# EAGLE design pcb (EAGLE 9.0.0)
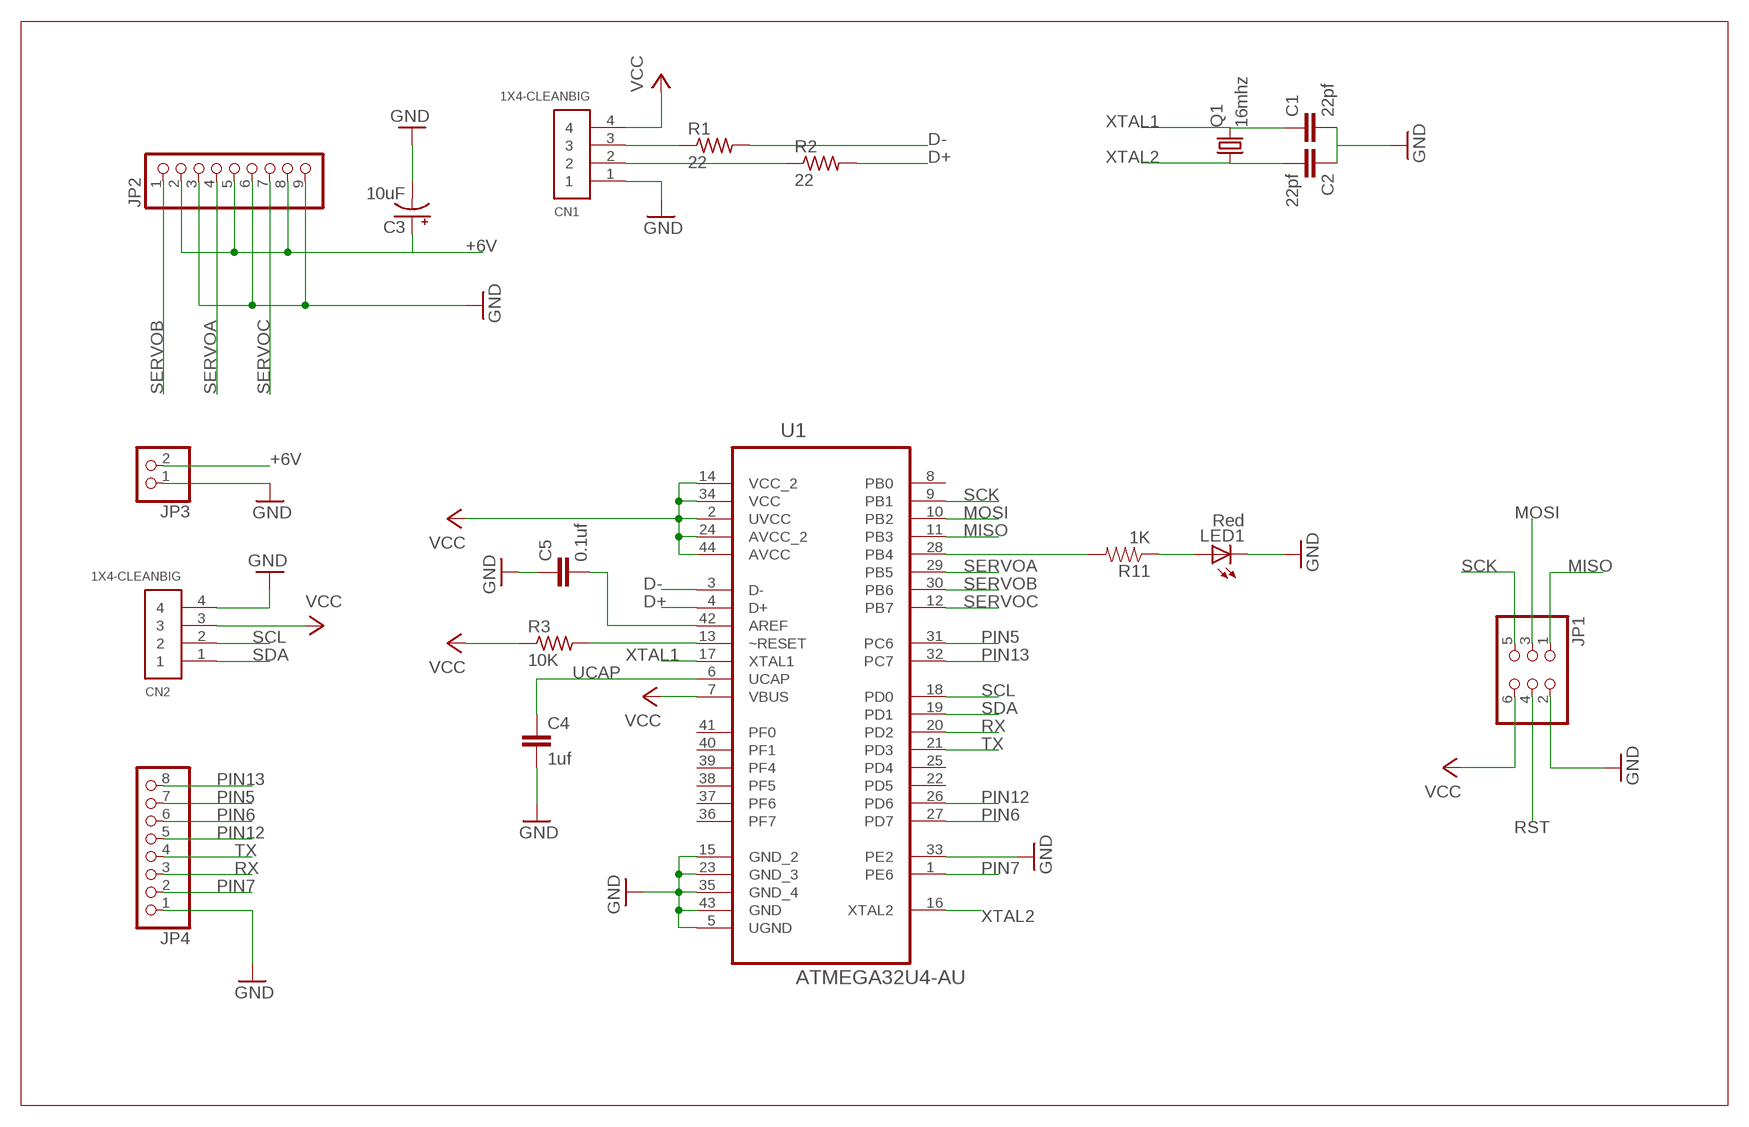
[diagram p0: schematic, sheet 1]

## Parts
C1  22pf  C5/2.5  [C5B2.5]
C2  22pf  C5/2.5  [C5B2.5]
C3  10uF  CAP_POL1206  [EIA3216]
C4  1uf  CC0603  [C0603]
C5  0.1uf  CC0603  [C0603]
CN1  1X4-CLEANBIG  [1X04-CLEANBIG]
CN2  1X4-CLEANBIG  [1X04-CLEANBIG]
JP1  PINHD-2X3  [2X03]
JP2  PINHD-1X9  [1X09-BIG]
JP3  PINHD-1X2  [1X02]
JP4  PINHD-1X8BIG  [1X08-BIG]
LED1  Red  LED0603  [LED-0603]
Q1  16mhz  CRYSTALHC49S  [HC49/S]
R1  22  R-US_R0603  [R0603]
R2  22  R-US_R0603  [R0603]
R3  10K  R-US_R0603  [R0603]
R11  1K  RESISTOR0603-RES  [0603-RES]
U1  ATMEGA32U4-AU  [QFP80P1200X1200X120-44N]

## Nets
+6V: C3.A(+) JP2.2 JP2.5 JP2.8 JP3.2
AREF: C5.2 U1.42(AREF)
D+: R2.2 U1.4(D+)
D-: R1.2 U1.3(D-)
GND: C1.2 C2.1 C3.C(-) C4.2 C5.1 CN1.1 CN2.4 JP1.2 JP2.3 JP2.6 JP2.9 JP3.1 JP4.1 LED1.C U1.5(UGND) U1.15(GND_2) U1.23(GND_3) U1.33(PE2) U1.35(GND_4) U1.43(GND)
MISO: JP1.1 U1.11(PB3)
MOSI: JP1.3 U1.10(PB2)
N$1: CN1.3 R1.1
N$2: CN1.2 R2.1
N$3: R11.2 U1.28(PB4)
N$4: LED1.A R11.1
PIN5: JP4.7 U1.31(PC6)
PIN6: JP4.6 U1.27(PD7)
PIN7: JP4.2 U1.1(PE6)
PIN12: JP4.5 U1.26(PD6)
PIN13: JP4.8 U1.32(PC7)
RST: JP1.4 R3.2 U1.13(~RESET)
RX: JP4.3 U1.20(PD2)
SCK: JP1.5 U1.9(PB1)
SCL: CN2.2 U1.18(PD0)
SDA: CN2.1 U1.19(PD1)
SERVOA: JP2.4 U1.29(PB5)
SERVOB: JP2.1 U1.30(PB6)
SERVOC: JP2.7 U1.12(PB7)
TX: JP4.4 U1.21(PD3)
UCAP: C4.1 U1.6(UCAP)
VCC: CN1.4 CN2.3 JP1.6 R3.1 U1.2(UVCC) U1.7(VBUS) U1.14(VCC_2) U1.24(AVCC_2) U1.34(VCC) U1.44(AVCC)
XTAL1: C1.1 Q1.2 U1.17(XTAL1)
XTAL2: C2.2 Q1.1 U1.16(XTAL2)
Unconnected: U1.8(PB0) U1.22(PD5) U1.25(PD4) U1.36(PF7) U1.37(PF6) U1.38(PF5) U1.39(PF4) U1.40(PF1) U1.41(PF0)

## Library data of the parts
C1 C2 = capacitor-wima:C: CAPACITOR
C3 = SparkFun:CAP_POL: Capacitor Polarized
C4 C5 = eagle-ltspice:C: CAPACITOR, European symbol; SPICEMODEL: NONE; SPICEPREFIX: C
CN1 CN2 = adafruit:1X4: 4-pin connector
JP1 = pinhead:PINHD-2X3: PIN HEADER
JP2 = adafruit:PINHD-1X9: Pin header 1x10 0.1" spacing With round pins
JP3 = pinhead:PINHD-1X2: PIN HEADER
JP4 = adafruit:PINHD-1X8: PIN HEADER
LED1 = SparkFun:LED: LEDs
Q1 = adafruit:CRYSTAL: CRYSTAL; OC_FARNELL: 1667008; OC_NEWARK: unknown
R1-R3 = adafruit:R-US_: RESISTOR, American symbol
R11 = SparkFun:RESISTOR: Resistor
U1 = ATMEGA32U4-AU:ATMEGA32U4-AU: 8-bit Microcontroller with ISP Flash and USB Controller; AVAILABILITY: Good; DESCRIPTION: MCU 8-bit ATmega AVR RISC 32KB Flash 3.3V/5V 44-Pin TQFP; MF: Microchip; MP: ATMEGA32U4-AU; PACKAGE: TQFP-44 Microchip; PRICE: 4.08 USD

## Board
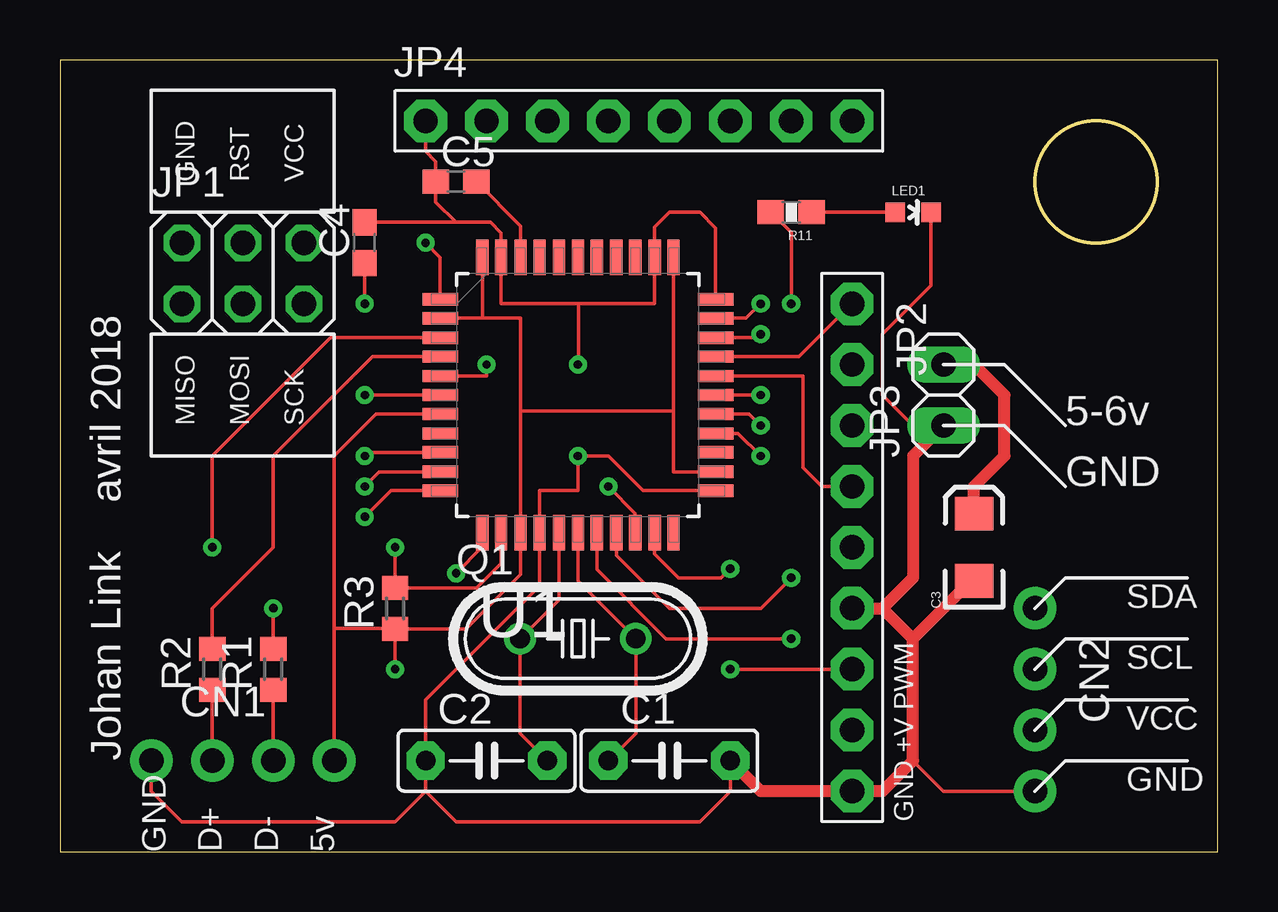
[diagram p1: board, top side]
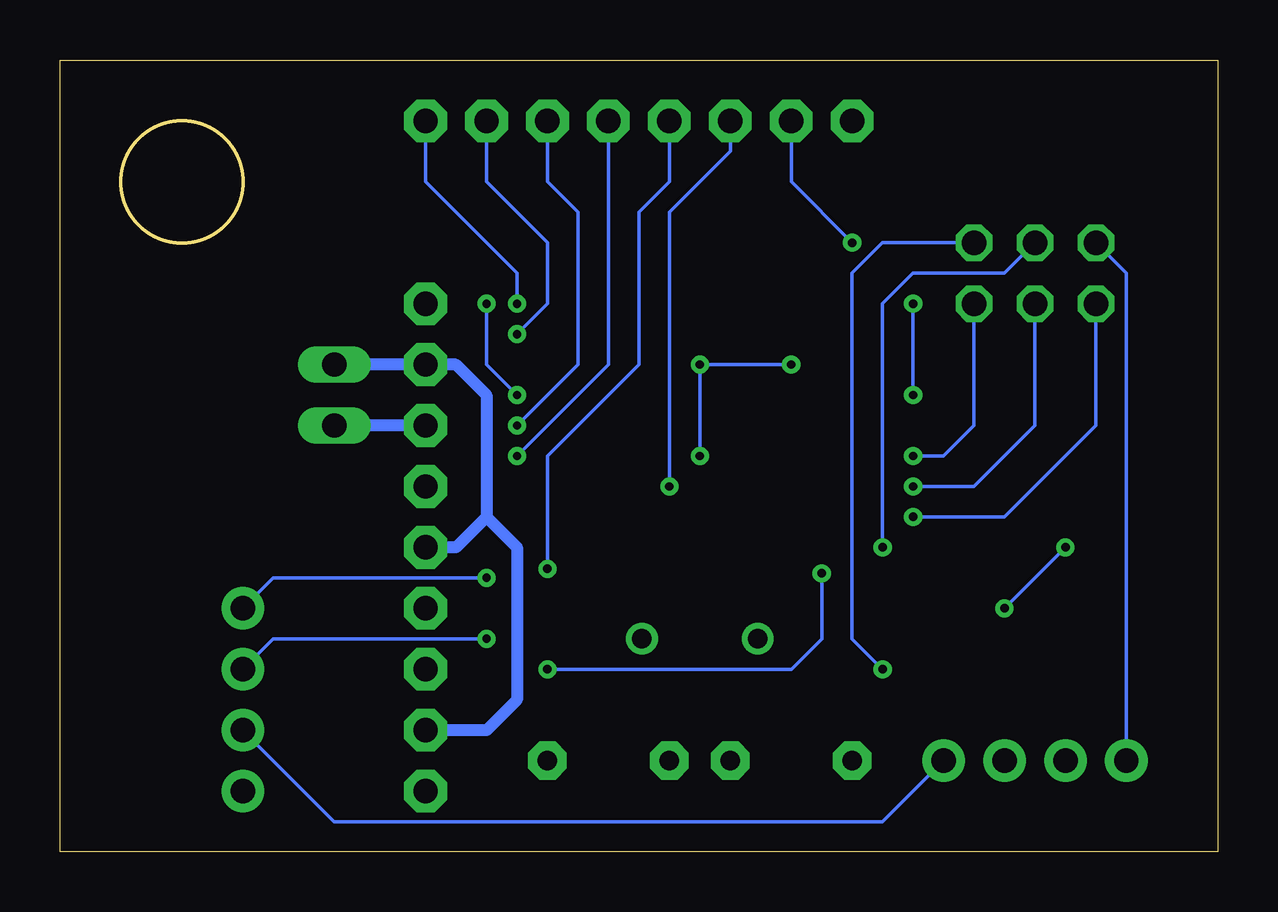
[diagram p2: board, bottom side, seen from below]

Size 48.26 x 33.02 mm. Coordinates in mm from the lower left corner, seen from the top.
Outline: 0,0 48.26,0 48.26,33.02 0,33.02 0,0
Outline: circle at 43.18,27.94 radius 2.54
Copper layers (1*16): Top 0.035mm / dielectric 1.5mm / Bottom 0.035mm
Design rules "default": minimum track width 6mil, minimum drill 0.35mm, track to track 6mil, track to pad 6mil, pad to pad 6mil, via to via 6mil, smd to smd 6mil, copper to edge 40mil, drill to drill 6mil, minimum pad ring 10mil, minimum via ring 8mil, stop-mask expansion 4mil, vias tented up to drill 0mil, thermal gap 10mil

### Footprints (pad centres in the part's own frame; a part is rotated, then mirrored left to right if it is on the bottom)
C5B2.5 = drill 0.813 pad 1.6 octagon: 1 -2.54,0; 2 2.54,0
EIA3216 = smd 1.4 x 1.6: A 1.4,0; C -1.4,0
C0603 = smd 1.1 x 1: 1 -0.85,0; 2 0.85,0
1X04-CLEANBIG = drill 1.016 pad 1.778: 1 -3.81,0; 2 -1.27,0; 3 1.27,0; 4 3.81,0
2X03 = drill 1.016 octagon: 1 -2.54,-1.27; 2 -2.54,1.27; 3 0,-1.27; 4 0,1.27; 5 2.54,-1.27; 6 2.54,1.27
1X09-BIG = drill 1.016 pad 1.778 octagon: 1 -10.16,0; 2 -7.62,0; 3 -5.08,0; 4 -2.54,0; 5 0,0; 6 2.54,0; 7 5.08,0; 8 7.62,0; 9 10.16,0
1X02 = drill 1.016 long: 1 -1.27,0; 2 1.27,0
1X08-BIG = drill 1.016 pad 1.778 octagon: 1 -8.89,0; 2 -6.35,0; 3 -3.81,0; 4 -1.27,0; 5 1.27,0; 6 3.81,0; 7 6.35,0; 8 8.89,0
LED-0603 = smd 0.8 x 0.8: A 0,-0.75; C 0,0.75
HC49/S = drill 0.813: 1 -2.413,0; 2 2.413,0
R0603 = smd 1 x 1.1: 1 -0.85,0; 2 0.85,0
0603-RES = smd 1.1 x 1: 1 -0.85,0; 2 0.85,0
QFP80P1200X1200X120-44N = smd 1.473 x 0.508: 1 -5.74,3.988; 2 -5.74,3.2; 3 -5.74,2.388; 4 -5.74,1.6; 5 -5.74,0.787; 6 -5.74,0; 7 -5.74,-0.787; 8 -5.74,-1.6; 9 -5.74,-2.388; 10 -5.74,-3.2; 11 -5.74,-3.988; 23 5.74,-3.988; 24 5.74,-3.2; 25 5.74,-2.388; 26 5.74,-1.6; 27 5.74,-0.787; 28 5.74,0; 29 5.74,0.787; 30 5.74,1.6; 31 5.74,2.388; 32 5.74,3.2; 33 5.74,3.988 | smd 0.508 x 1.473: 12 -3.988,-5.74; 13 -3.2,-5.74; 14 -2.388,-5.74; 15 -1.6,-5.74; 16 -0.787,-5.74; 17 0,-5.74; 18 0.787,-5.74; 19 1.6,-5.74; 20 2.388,-5.74; 21 3.2,-5.74; 22 3.988,-5.74; 34 3.988,5.74; 35 3.2,5.74; 36 2.388,5.74; 37 1.6,5.74; 38 0.787,5.74; 39 0,5.74; 40 -0.787,5.74; 41 -1.6,5.74; 42 -2.388,5.74; 43 -3.2,5.74; 44 -3.988,5.74

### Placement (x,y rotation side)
C1  25.4,3.81 0 top
C2  17.78,3.81 0 top
C3  38.1,12.7 90 top
C4  12.7,25.4 90 top
C5  16.51,27.94 0 top
CN1  7.62,3.81 0 top
CN2  40.64,6.35 270 top
JP1  7.62,24.13 0 top
JP2  33.02,12.7 270 top
JP3  36.83,19.05 90 top
JP4  24.13,30.48 0 top
LED1  35.56,26.67 270 top
Q1  21.59,8.89 0 top
R1  8.89,7.62 90 top
R2  6.35,7.62 90 top
R3  13.97,10.16 90 top
R11  30.48,26.67 180 top
U1  21.59,19.05 0 top

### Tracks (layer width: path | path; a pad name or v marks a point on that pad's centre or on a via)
+6V
  Top 0.508: C3.A 38.1,15.24 39.37,16.51 39.37,19.05 38.1,20.32 JP3.2
  Bottom 0.508: 30.48,13.97 30.48,19.05 31.75,20.32 JP2.2 JP3.2 | 30.48,13.97 29.21,12.7 29.21,6.35 30.48,5.08 JP2.8 | 30.48,13.97 31.75,12.7 JP2.5
AREF
  Top 0.152: C5.2 19.2,26.1 U1.42
D+
  Top 0.152: U1.4 13.03,20.65 8.89,16.51 8.89,12.7 6.35,10.16 R2.2
D-  (via drill 0.35)
  Top 0.152: U1.3 11.28,21.44 6.35,16.51 v6.35,12.7 | R1.2 v8.89,10.16
  Bottom 0.152: v8.89,10.16 v6.35,12.7
GND  (via drill 0.35)
  Top 0.152: 21.61,22.86 24.79,22.86 U1.35 24.79,26.06 25.4,26.67 26.67,26.67 27.33,26.01 U1.33 | 21.61,22.86 18.39,22.86 U1.43 18.39,25.81 17.95,26.25 16.51,26.25 | U1.5 17.78,19.84 v17.78,20.32 | v21.59,20.32 21.61,20.32 21.61,22.86 | 15.24,2.54 C2.1 15.24,6.35 19.99,11.1 U1.15 19.99,15.06 21.59,15.06 v21.59,16.51 22.86,16.51 24.31,15.06 U1.23 | 15.24,2.54 16.51,1.27 26.67,1.27 27.94,2.54 C1.2 | CN1.1 3.81,2.54 5.08,1.27 13.97,1.27 15.24,2.54 | CN2.4 36.83,2.54 35.56,3.81 | LED1.C 36.31,23.61 34.29,21.59 34.29,19.05 35.56,17.78 JP3.1 | C4.2 16.51,26.25 | 16.51,26.25 15.66,27.1 C5.1 15.66,28.79 15.24,29.21 JP4.1
  Top 0.508: JP2.6 34.29,10.16 | 34.29,10.16 35.56,11.43 35.56,16.51 JP3.1 | 35.56,8.89 34.29,10.16 | 35.56,8.89 35.56,3.81 34.29,2.54 JP2.9 29.21,2.54 C1.2 | C3.C 37.97,11.3 35.56,8.89
  Bottom 0.152: v17.78,20.32 v21.59,20.32 v21.59,16.51 | JP1.2 3.81,24.13 CN1.1
  Bottom 0.508: JP2.3 JP3.1
MISO  (via drill 0.35)
  Top 0.152: U1.11 13.79,15.06 v12.7,13.97
  Bottom 0.152: v12.7,13.97 8.89,13.97 5.08,17.78 JP1.1
MOSI  (via drill 0.35)
  Top 0.152: U1.10 13.31,15.85 v12.7,15.24
  Bottom 0.152: v12.7,15.24 10.16,15.24 7.62,17.78 JP1.3
N$1
  Top 0.152: R1.1 CN1.3
N$2
  Top 0.152: R2.1 CN1.2
N$3  (via drill 0.35)
  Top 0.152: U1.28 v29.21,19.05 | R11.2 30.48,25.82 v30.48,22.86
  Bottom 0.152: v29.21,19.05 30.48,20.32 v30.48,22.86
N$4
  Top 0.152: R11.1 LED1.A
PIN5  (via drill 0.35)
  Top 0.152: U1.31 29.06,21.44 v29.21,21.59
  Bottom 0.152: v29.21,21.59 27.94,22.86 27.94,25.4 30.48,27.94 JP4.7
PIN6  (via drill 0.35)
  Top 0.152: v29.21,17.78 28.73,18.26 U1.27
  Bottom 0.152: v29.21,17.78 26.67,20.32 26.67,26.67 27.94,27.94 JP4.6
PIN7  (via drill 0.35)
  Top 0.152: U1.1 15.85,24.79 v15.24,25.4
  Bottom 0.152: v15.24,25.4 17.78,27.94 JP4.2
PIN12  (via drill 0.35)
  Top 0.152: U1.26 28.27,17.45 v29.21,16.51
  Bottom 0.152: v29.21,16.51 25.4,20.32 JP4.5
PIN13  (via drill 0.35)
  Top 0.152: U1.32 28.6,22.25 v29.21,22.86
  Bottom 0.152: v29.21,22.86 29.21,24.13 33.02,27.94 JP4.8
RST  (via drill 0.35)
  Top 0.152: U1.13 18.39,12.04 17.36,11.01 R3.2 v13.97,12.7
  Bottom 0.152: v13.97,12.7 13.97,22.86 12.7,24.13 8.89,24.13 JP1.4
RX  (via drill 0.35)
  Top 0.152: U1.20 23.98,14.12 v22.86,15.24
  Bottom 0.152: v22.86,15.24 22.86,26.67 20.32,29.21 JP4.3
SCK  (via drill 0.35)
  Top 0.152: U1.9 12.85,16.66 v12.7,16.51
  Bottom 0.152: v12.7,16.51 11.43,16.51 10.16,17.78 JP1.5
SCL  (via drill 0.35)
  Top 0.152: U1.18 22.38,11.77 25.26,8.89 v30.48,8.89
  Bottom 0.152: v30.48,8.89 39.37,8.89 CN2.2
SDA  (via drill 0.35)
  Top 0.152: U1.19 23.19,12.37 25.4,10.16 29.21,10.16 v30.48,11.43
  Bottom 0.152: v30.48,11.43 39.37,11.43 CN2.1
SERVOA
  Top 0.152: U1.29 30.96,19.84 30.96,16.03 31.75,15.24 JP2.4
SERVOB
  Top 0.152: U1.30 30.81,20.65 JP2.1
SERVOC  (via drill 0.35)
  Top 0.152: U1.12 17.6,12.71 v16.51,11.62 | v27.94,7.62 JP2.7
  Bottom 0.152: v16.51,11.62 16.51,8.89 17.78,7.62 v27.94,7.62
TX  (via drill 0.35)
  Top 0.152: U1.21 24.79,12.42 25.78,11.43 27.56,11.43 v27.94,11.81
  Bottom 0.152: v27.94,11.81 27.94,16.51 24.13,20.32 24.13,26.67 22.86,27.94 JP4.4
UCAP  (via drill 0.35)
  Top 0.152: U1.6 v12.7,19.05 | v12.7,22.86 C4.1
  Bottom 0.152: v12.7,19.05 v12.7,22.86
VCC  (via drill 0.35)
  Top 0.152: 25.58,18.39 19.2,18.39 | 19.2,18.39 U1.14 19.2,11.58 16.93,9.31 R3.1 | 17.61,22.25 U1.2 | 17.61,22.25 19.2,22.25 19.2,18.39 | U1.44 17.61,24.79 17.61,22.25 | U1.24 25.58,15.85 25.58,18.39 | U1.34 25.58,18.39 | v13.97,7.62 R3.1 | 11.43,9.32 CN1.4 | 11.43,9.32 11.43,16.51 13.18,18.26 U1.7 | R3.1 13.96,9.32 11.43,9.32
  Bottom 0.152: JP1.6 13.97,25.4 15.24,24.13 15.24,8.89 v13.97,7.62 | CN2.3 36.83,1.27 13.97,1.27 CN1.4
XTAL1
  Top 0.152: C1.1 24,4.95 Q1.2 21.59,11.3 U1.17
XTAL2
  Top 0.152: C2.2 19.18,4.95 Q1.1 20.8,10.52 U1.16

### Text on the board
tPlace: GND / / RST / / VCC | MISO / / MOSI / / SCK | 5-6v | GND | SDA | SCL | VCC | Johan Link avril 2018 | GND | GND +V PWM | GND / D+ / D- / 5v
